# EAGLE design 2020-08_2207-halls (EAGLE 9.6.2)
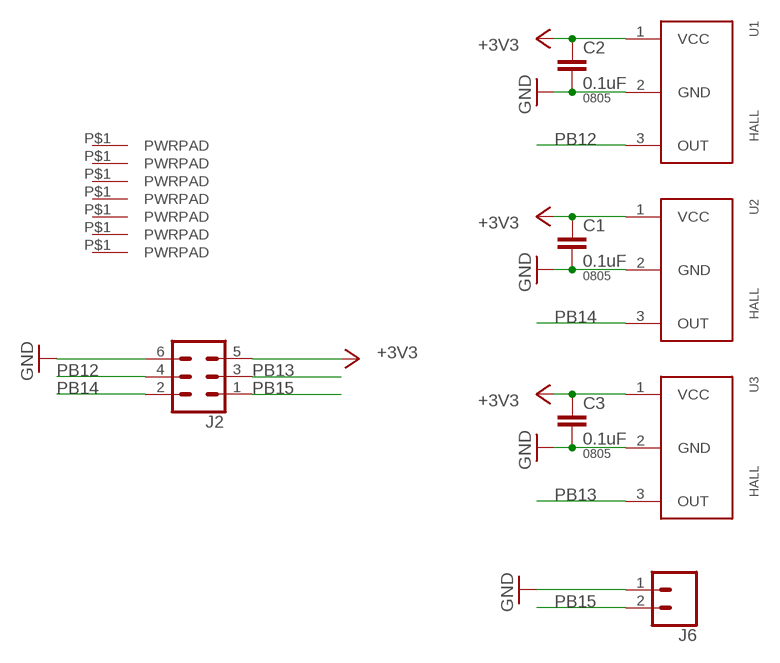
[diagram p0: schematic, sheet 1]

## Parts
C1  0.1uF  CAP0805  [0805]
C2  0.1uF  CAP0805  [0805]
C3  0.1uF  CAP0805  [0805]
J1  PWRPADM3-SKINNY  [PWRPAD_3-25MM-SKINNY]
J2  CONN_03X2SHROUD  [2X3-SHROUDED]
J3  PWRPADM3-SKINNY  [PWRPAD_3-25MM-SKINNY]
J4  PWRPADM3-SKINNY  [PWRPAD_3-25MM-SKINNY]
J5  PWRPADM3-SKINNY  [PWRPAD_3-25MM-SKINNY]
J6  CONN_02LOCK  [1X02_LOCK]
J7  PWRPADM3-SKINNY  [PWRPAD_3-25MM-SKINNY]
J8  PWRPADM3-SKINNY  [PWRPAD_3-25MM-SKINNY]
J9  PWRPADM3-SKINNY  [PWRPAD_3-25MM-SKINNY]
U1  HALL  [TO-92-AMMO]
U2  HALL  [TO-92-AMMO]
U3  HALL  [TO-92-AMMO]

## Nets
+3V3: C1.1 C2.1 C3.1 J2.5 U1.1(VCC) U2.1(VCC) U3.1(VCC)
GND: C1.2 C2.2 C3.2 J2.6 J6.1 U1.2(GND) U2.2(GND) U3.2(GND)
PB12: J2.4 U1.3(OUT)
PB13: J2.3 U3.3(OUT)
PB14: J2.2 U2.3(OUT)
PB15: J2.1 J6.2
Unconnected: J1.P$1(PWRPAD) J3.P$1(PWRPAD) J4.P$1(PWRPAD) J5.P$1(PWRPAD) J7.P$1(PWRPAD) J8.P$1(PWRPAD) J9.P$1(PWRPAD)

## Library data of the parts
C1-C3 = passives:CAP: Capacitor; PACKAGE: 0805
J1 J3-J5 J7-J9 = connector:PWRPAD
J2 = SparkFun-Connectors:CONN_03X2: Multi connection point. Often used as Generic Header-pin footprint for 0.1 inch spaced/style header connections You can populate with any combo of single row headers, but if you'd like an exact match, check these: Header - 2x3 (Male, 0.1") (PRT-12807) Header - 2x3 (Female, 0.1") (PRT-13010) 2x3 Pin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; PROD_ID: CONN-10681; SF_ID: PRT_10877
J6 = SparkFun-Connectors:CONN_02: Multi connection point. Often used as Generic Header-pin footprint for 0.1 inch spaced/style header connections
U1-U3 = sensor:HALL

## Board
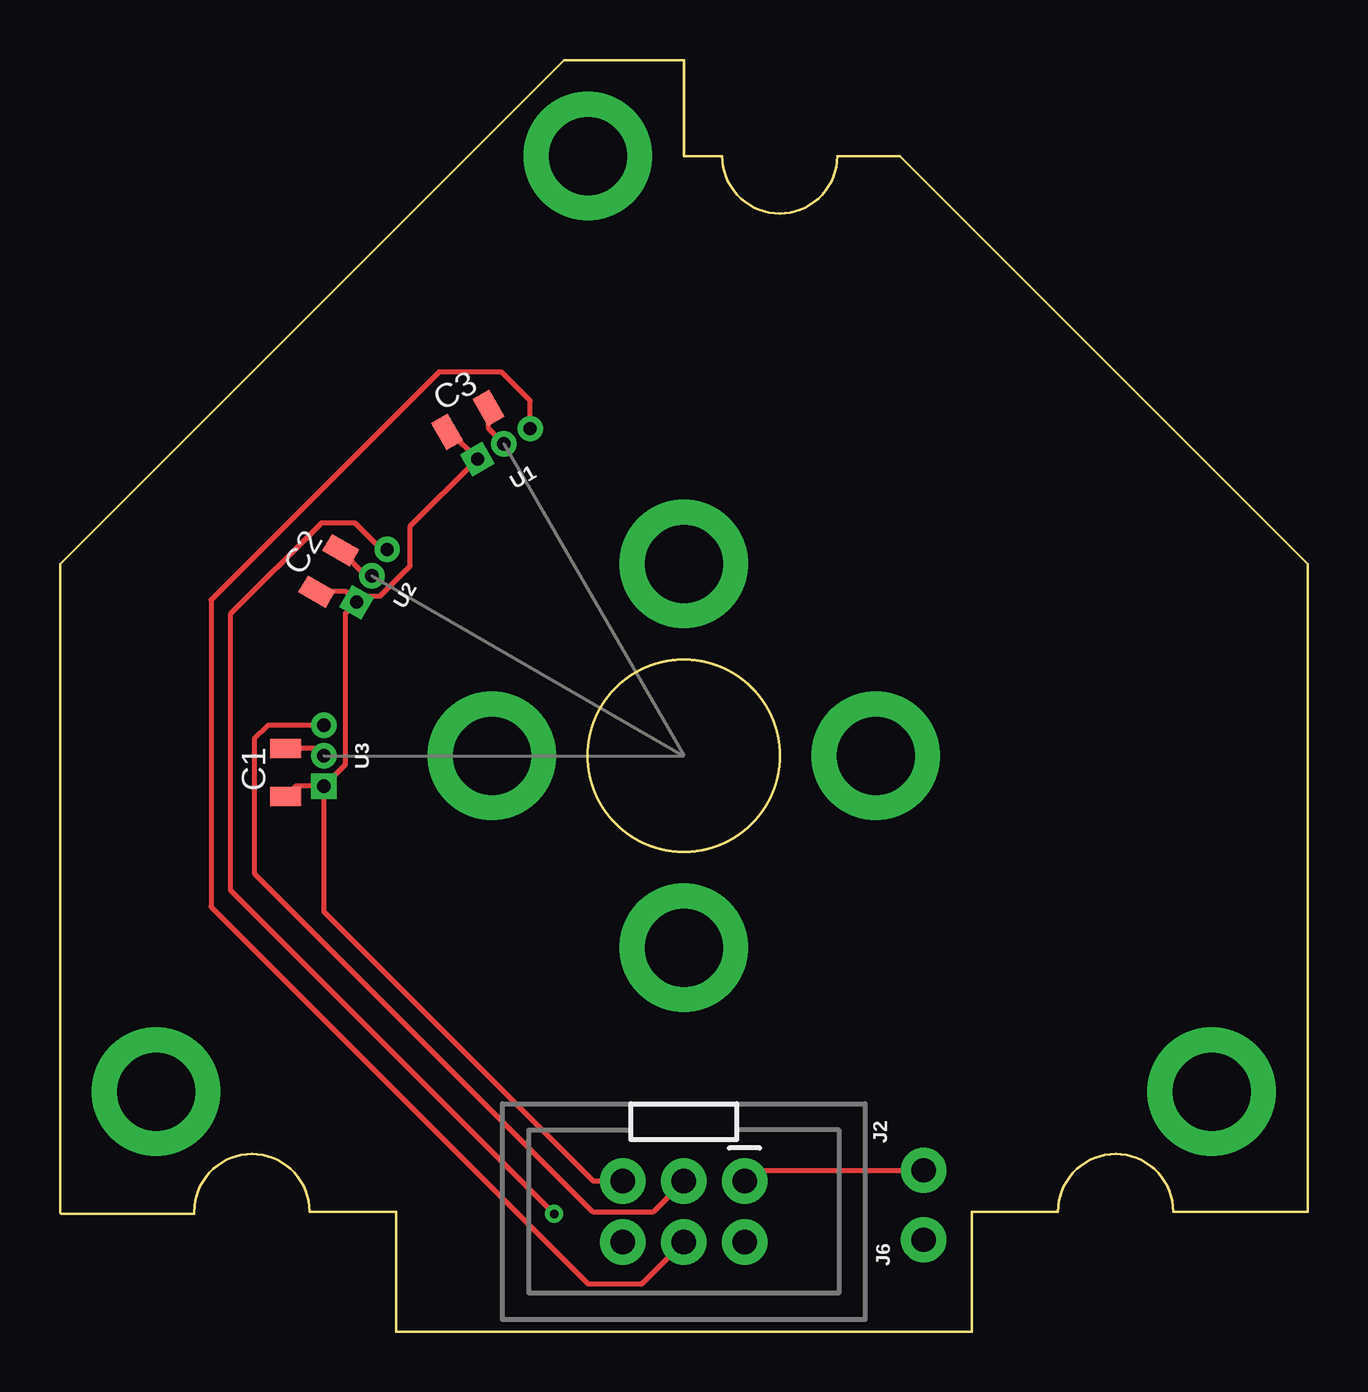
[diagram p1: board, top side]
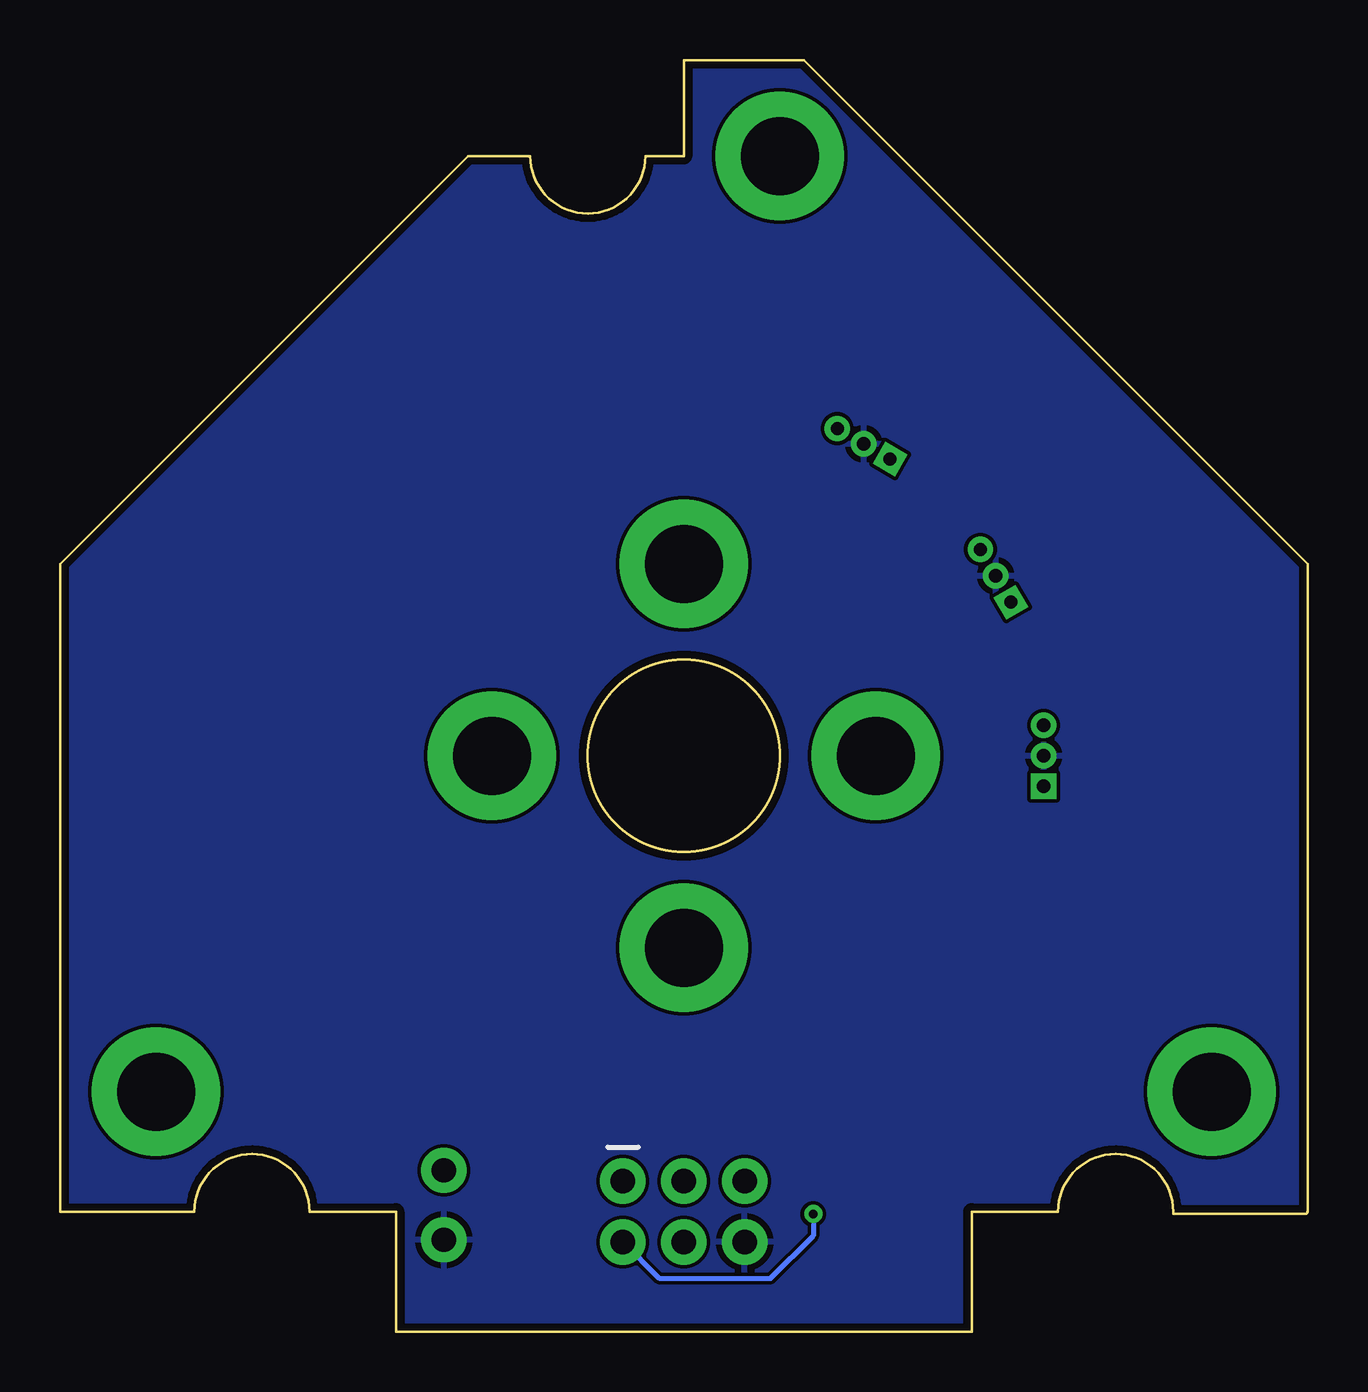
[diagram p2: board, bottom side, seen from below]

Size 52 x 53 mm. Coordinates in mm from the lower left corner, seen from the top.
Outline: 35,49 52,32 52,5 46.4,5 arc90 44,7.4 arc90 41.6,5 38,5 38,0 14,0 14,5 10.4,5 arc90 8,7.4 arc90 5.6,5 5.6,4.9 0.1,4.9 arc-90 0,5 0,32 21,53 26,53 26,49 27.6,49 arc90 30,46.6 arc90 32.4,49 35,49
Outline: circle at 26,24 radius 4
Copper layers (1*16): Top 0.035mm / dielectric 1.5mm / Bottom 0.035mm
Design rules "default *": minimum track width 6mil, minimum drill 0.35mm, track to track 6mil, track to pad 6mil, pad to pad 6mil, via to via 6mil, smd to smd 6mil, copper to edge 12mil, drill to drill 6mil, minimum pad ring 10mil, minimum via ring 8mil, stop-mask expansion 4mil, vias tented up to drill 35mil, thermal gap 10mil

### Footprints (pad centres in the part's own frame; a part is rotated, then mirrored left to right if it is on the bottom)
0805 = smd 0.8 x 1.3: 1 -1,0; 2 1,0
PWRPAD_3-25MM-SKINNY = drill 3.25 pad 5.35: P$1 0,0
2X3-SHROUDED = drill 1.016 pad 1.88: 1 -1.27,2.54; 2 1.27,2.54; 3 -1.27,0; 4 1.27,0; 5 -1.27,-2.54; 6 1.27,-2.54
1X02_LOCK = drill 1.016 pad 1.88: 1 -0.178,0; 2 2.718,0
TO-92-AMMO = drill 0.55 square: 1 -1.27,0 | drill 0.55: 2 0,0; 3 1.27,0

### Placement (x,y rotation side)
C1  9.4,23.3 90 top
C2  11.2,31.7 60 top
C3  17,38 30 top
J1  26,16 0 top
J2  26,5 270 top
J3  26,32 0 top
J4  34,24 0 top
J5  18,24 0 top
J6  36,4 90 top
J7  4,10 0 top
J8  48,10 0 top
J9  22,49 0 top
U1  18.5,37 30 top
U2  13,31.5 60 top
U3  11,24 90 top

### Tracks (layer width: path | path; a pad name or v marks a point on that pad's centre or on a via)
+3V3
  Top 0.203: C3.1 16.27,37.5 U1.1 14.6,33.56 14.6,31.91 13.35,30.66 12.62,30.66 U2.1 | U2.1 11.93,30.83 C2.1 | U3.1 9.83,22.73 C1.1 | J2.5 22.23,6.27 11,17.5 U3.1 | U3.1 11.9,23.63 11.9,29.93 U2.1
GND
  Top 0.203: U2.2 12.77,31.5 C2.2 | U1.2 17.87,37.63 C3.2 | U3.2 10.7,24.3 C1.2
  pour Bottom: -1,-1 -1,54 53,54 53,-1
PB12
  Top 0.203: U1.3 19.6,38.8 18.4,40 15.8,40 6.3,30.5 6.3,17.7 22,2 24.27,2 J2.4
PB13
  Top 0.203: U3.3 8.67,25.27 8.1,24.7 8.1,19.1 22.2,5 24.73,5 J2.3
PB14  (via drill 0.35)
  Top 0.203: U2.3 13.4,32.6 12.3,33.7 10.9,33.7 7.1,29.9 7.1,18.4 v20.6,4.9
  Bottom 0.203: v20.6,4.9 20.6,4 22.4,2.2 27.01,2.2 J2.2
PB15
  Top 0.203: J2.1 28.99,6.72 J6.2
